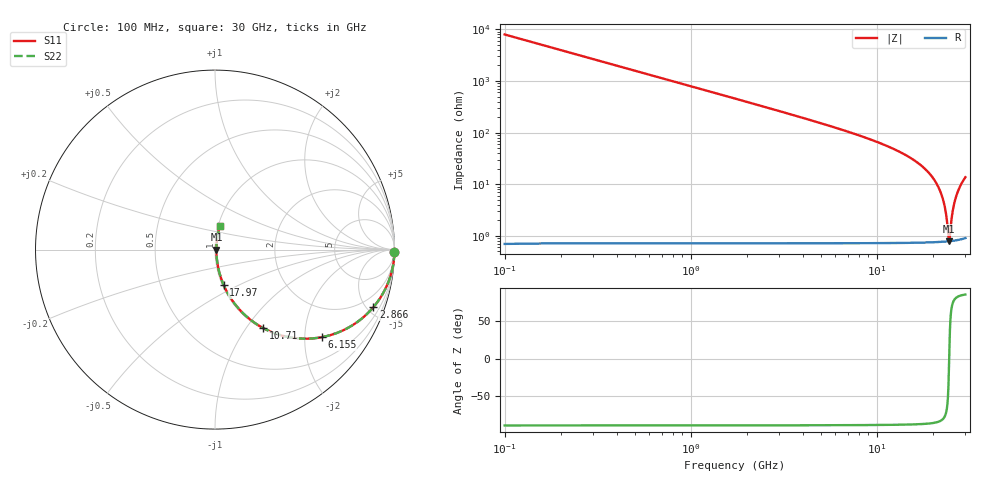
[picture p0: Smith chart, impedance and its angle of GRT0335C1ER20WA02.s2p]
!Murata Part Number: GRT0335C1ER20WA02
!These Parameters are Measured in Series Mode Connection
!Data Generated on Jun 19, 2026
!  o--ll--o
!Port1  Port2
!  o------o
!Operation Temp=25[degC], DC Bias Voltage=0[V]
!Freq. Start=100[MHz] Stop=30[GHz] 401[Steps]
# Hz S RI R 50
!Freq.(Hz) S11(Real) S11(Imag) S21(Real) S21(Imag) S12(Real) S12(Imag) S22(Real) S22(Imag)
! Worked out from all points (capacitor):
!   401 points, 100 MHz to 30 GHz, reference 50 ohm
!   read as one part in series: C = 200 fF near 249.5 MHz
!   lowest |Z| = 790 mohm at 24.54 GHz (marker M1)
!   series resonance near 24.54 GHz, so ESL is about 210 pH
!   S11 on the Smith chart (normalised r, x): 100 MHz: open; 2.866 GHz: 1.01, -5.48; 6.155 GHz: 1.01, -2.43; 10.71 GHz: 1.01, -1.21; 17.97 GHz: 1.01, -0.41; 30 GHz: 1.02, +0.27
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1e8  0.9998 -0.0126  0.000159 0.0126  0.000159 0.0126  0.9998 -0.0126
4.7375e8  0.9964 -0.0593  0.00356 0.0593  0.00356 0.0593  0.9964 -0.0593
9.2225e8  0.9866 -0.1145  0.0134 0.1145  0.0134 0.1145  0.9866 -0.1145
1.7445e9  0.9534 -0.21  0.0466 0.21  0.0466 0.21  0.9534 -0.21
2.86575e9  0.8818 -0.3216  0.1182 0.3216  0.1182 0.3216  0.8818 -0.3216
5.10825e9  0.689 -0.4605  0.311 0.4605  0.311 0.4605  0.689 -0.4605
6.15475e9  0.5947 -0.488  0.4053 0.488  0.4053 0.488  0.5947 -0.488
1.01165e10  0.302 -0.4536  0.698 0.4536  0.698 0.4536  0.302 -0.4536
1.07145e10  0.269 -0.4375  0.731 0.4375  0.731 0.4375  0.269 -0.4375
1.505e10  0.1045 -0.295  0.8955 0.295  0.8955 0.295  0.1045 -0.295
1.796525e10  0.0477 -0.196  0.9523 0.196  0.9523 0.196  0.0477 -0.196
2.005825e10  0.0245 -0.129  0.9755 0.129  0.9755 0.129  0.0245 -0.129
2.170275e10  0.014 -0.0793  0.986 0.0793  0.986 0.0793  0.014 -0.0793
2.289875e10  0.00971 -0.0449  0.9903 0.0449  0.9903 0.0449  0.00971 -0.0449
2.364625e10  0.00833 -0.0241  0.9917 0.0241  0.9917 0.0241  0.00833 -0.0241
2.439375e10  0.00784 -0.00387  0.9922 0.00387  0.9922 0.00387  0.00784 -0.00387
2.454325e10  0.00784 0.000112  0.9922 -0.000112  0.9922 -0.000112  0.00784 0.000112
2.50665e10  0.0081 0.0139  0.9919 -0.0139  0.9919 -0.0139  0.0081 0.0139
2.573925e10  0.00898 0.0312  0.991 -0.0312  0.991 -0.0312  0.00898 0.0312
2.6711e10  0.0113 0.0555  0.9887 -0.0555  0.9887 -0.0555  0.0113 0.0555
2.813125e10  0.0166 0.0895  0.9834 -0.0895  0.9834 -0.0895  0.0166 0.0895
3e10  0.0269 0.1318  0.9731 -0.1318  0.9731 -0.1318  0.0269 0.1318
